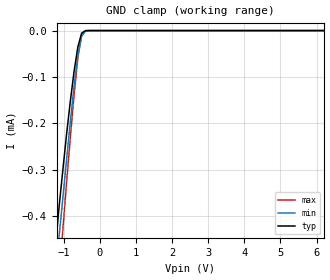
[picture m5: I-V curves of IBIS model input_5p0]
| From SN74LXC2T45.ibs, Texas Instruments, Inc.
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|   input_5p0 Model
[Model]   input_5p0
Model_type   Input
Vinl = 2.0
Vinh = 3.0
|   typ   min   max
C_comp   2.81pF   2.18pF   3.98pF
[Voltage Range]   5   4.5   5.5
|Junction Temperature
[Temperature Range]   25   125   -40
[GND Clamp Reference]   0   0   0
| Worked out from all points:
|   GND clamp passes 1 mA (typ) near -1.81 V on its own axis
[GND Clamp]
|   Voltage   I(typ)   I(min)   I(max)
-2.5V     -1.66mA    -1.64mA    -2.09mA
-1.24V    -478uA     -541uA     -650uA
-1.14V    -389uA     -453uA     -542uA
-1.03V    -305uA     -366uA     -435uA
-925mV    -226uA     -281uA     -332uA
-820mV    -154uA     -198uA     -233uA
-715mV    -88.7uA    -121uA     -140uA
-610mV    -35.6uA    -55uA      -59.7uA
-505mV    -5.5uA     -12.7uA    -8.49uA
-400mV    -210nA     -1.14uA    -141nA
8V        3.62nA     3.43nA     4.22nA
